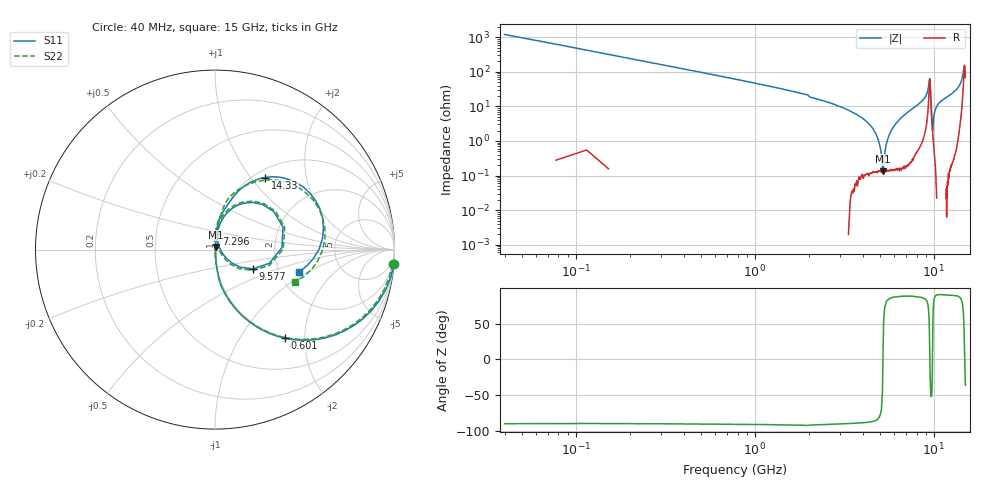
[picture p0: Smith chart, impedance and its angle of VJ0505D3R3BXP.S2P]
! VJ0505D3R3BXP
! MLCC placed on 25 mil thick microstrip substrate in series configuraton.
! DATE 06/29/2018  07:46
! CORRECTED  DATA
# GHz  S  MA  R  50.00
!  FREQ  S11M  S11A  S21M  S21A  S12M  S12A  S22M  S22A
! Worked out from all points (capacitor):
!   401 points, 40 MHz to 15 GHz, reference 50 ohm
!   read as one part in series: C = 3.28 pF near 114.8 MHz
!   lowest |Z| = 133 mohm at 5.201 GHz (marker M1)
!   series resonance near 5.195 GHz, so ESL is about 290 pH
!   S11 on the Smith chart (normalised r, x): 40 MHz: -0, -25; 601 MHz: 0.98, -1.60; 7.296 GHz: 1.00, +0.18; 9.577 GHz: 1.49, -0.34; 14.33 GHz: 1.12, +1.18; 15 GHz: 2.56, -0.84
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0.04  1 -4.7  0.08333 85.5  0.08264 85.8  0.9932 -4.7
0.2644  0.8823 -28.6  0.4798 61.6  0.4802 61.7  0.875 -28.5
0.601  0.6294 -51.7  0.7864 39.1  0.7871 39.1  0.6246 -51.6
2.5458  0.1237 -83.4  0.994 8.1  0.9943 8.1  0.1237 -83.4
4.154  0.02589 -81.0  0.9981 2.9  0.9984 3.0  0.02537 -90.1
4.4906  0.01227 -72.8  0.9981 2.2  0.9987 2.3  0.01162 -96.3
4.7898  0.003354 -0.1  0.9979 1.6  0.9985 1.6  0.001651 172.0
5.0516  0.01027 70.5  0.998 1.1  0.9983 1.2  0.00989 100.7
5.2012  0.01567 77.1  0.9979 0.8  0.9985 0.9  0.01525 97.6
5.9492  0.04259 83.7  0.9971 -0.5  0.9978 -0.5  0.04228 92.2
7.2956  0.08901 83.6  0.9931 -3.2  0.9936 -3.2  0.09074 87.9
7.52  0.09826 82.9  0.9917 -3.7  0.9926 -3.7  0.1003 87.1
9.3152  0.3096 57.0  0.8606 -15.6  0.8614 -15.6  0.3174 57.4
9.4648  0.3993 18.5  0.6236 -8.6  0.624 -8.6  0.4076 17.7
9.577  0.2368 -26.9  0.8018 10.4  0.8024 10.4  0.2404 -28.9
9.8014  0.02763 20.6  0.9769 1.4  0.9775 1.4  0.02012 22.1
10.0258  0.07193 81.2  0.9908 -2.2  0.9917 -2.2  0.0726 85.9
10.6242  0.1344 83.4  0.9914 -5.9  0.992 -5.9  0.1371 85.6
12.5316  0.231 76.5  0.9693 -12.0  0.9702 -12.0  0.239 78.7
14.3268  0.4884 55.3  0.8026 -27.9  0.8033 -27.9  0.4926 52.0
14.7382  0.6272 21.8  0.4481 -24.3  0.4483 -24.3  0.625 16.0
15  0.4837 -15.0  0.5702 17.4  0.5708 17.4  0.4784 -22.1
